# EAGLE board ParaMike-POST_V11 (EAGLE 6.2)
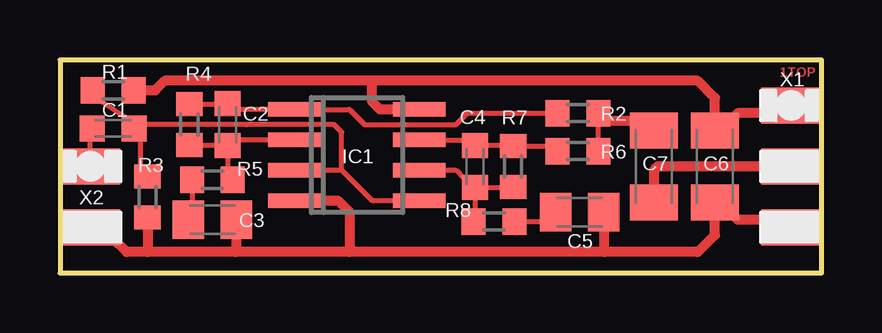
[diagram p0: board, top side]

Size 31.75 x 8.89 mm. Coordinates in mm from the lower left corner, seen from the top.
Outline: 0,8.89 0,0 31.75,0 31.75,8.89 0,8.89
Copper layers (1*16): Top 0.035mm / dielectric 1.5mm / Bottom 0.035mm
Design rules: minimum track width 6mil, minimum drill 12mil, track to track 6mil, track to pad 6mil, pad to pad 6mil, via to via 6mil, smd to smd 6mil, copper to edge 20mil, drill to drill 8mil, minimum pad ring 8mil, minimum via ring 6mil, stop-mask expansion 3mil, vias tented up to drill 0mil, thermal gap 8mil

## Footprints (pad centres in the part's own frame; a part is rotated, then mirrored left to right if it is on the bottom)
C0603K = smd 1.05 x 1.08: 1 -0.875,0; 2 0.875,0
C0805K = smd 1.3 x 1.6: 1 -1,0; 2 1,0
C1206K = smd 1.5 x 2: 1 -1.5,0; 2 1.5,0
SO08 = smd 0.6 x 2.2: 1 -1.905,-2.6; 2 -0.635,-2.6; 3 0.635,-2.6; 4 1.905,-2.6; 5 1.905,2.6; 6 0.635,2.6; 7 -0.635,2.6; 8 -1.905,2.6
R0603 = smd 1 x 1.1: 1 -0.85,0; 2 0.85,0
AKK3PAD-HALF = smd 2.5 x 1.5: 1 0,2.54; 2 0,0; 3 0,-2.54
AKK2PAD-HALF = smd 2.5 x 1.5: 1 0,1.27; 2 0,-1.27

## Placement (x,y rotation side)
C1  22n  [C0603K]  2.22,6.03 0 top
C2  1n  [C0603K]  6.99,6.19 270 top
C3  220n  [C0805K]  6.35,2.22 0 top
C4  1n  [C0603K]  17.3,4.45 270 top
C5  220n  [C0805K]  21.67,2.54 0 top
C6  22u;10V  [C1206K]  27.3,4.45 270 top
C7  22u;10V  [C1206K]  24.77,4.45 270 top
IC1  NJM4556  [SO08]  12.38,4.92 270 top
R1  47k  [R0603]  2.22,7.62 0 top
R2  10E  [R0603]  21.59,6.67 180 top
R3  47k  [R0603]  3.65,3.17 90 top
R4  22k  [R0603]  5.4,6.19 90 top
R5  2k2  [R0603]  6.35,3.89 0 top
R6  10E  [R0603]  21.59,5.08 180 top
R7  22k  [R0603]  18.89,4.45 90 top
R8  2k2  [R0603]  18.1,2.14 180 top
X1  AKK3PAD-HALF  [AKK3PAD-HALF]  30.48,4.45 0 top
X2  AKK2PAD-HALF  [AKK2PAD-HALF]  1.27,3.17 0 top

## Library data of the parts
C1 C2 C4 R1-R8 = rcl
C3 C5 = rcl; SIZE: 0805
C6 C7 = rcl; SIZE: 1206
IC1 = linear
X1 X2 = Akki_V6

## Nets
+BAT: C6.1 IC1.8 R1.2 X1.1
GND: C3.2 C5.2 C6.2 IC1.4 R3.1 X1.3 X2.2
N$1: C3.1 R5.1
N$2: C1.2 IC1.3 IC1.5 R1.1 R3.2
N$3: C2.2 IC1.2 R4.1 R5.2
N$4: C2.1 IC1.1 R2.2 R4.2
N$5: C7.2 X1.2
N$6: C1.1 X2.1
N$7: C7.1 R2.1 R6.1
N$8: C4.2 IC1.6 R7.1 R8.2
N$9: C4.1 IC1.7 R6.2 R7.2
N$10: C5.1 R8.1

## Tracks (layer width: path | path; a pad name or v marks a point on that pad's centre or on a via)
+BAT
  Top 0.406: X1.1 29.84,6.99 29.53,6.67 28.26,6.67 27.94,6.35 27.71,6.35 C6.1 27.3,7.3 26.59,8.02 13.02,8.02 | 13.02,8.02 4.37,8.02 3.97,7.62 R1.2 | IC1.8 13.34,6.83 13.02,7.14 13.02,8.02
GND
  Top 0.406: X1.3 30,1.91 29.53,1.43 29.53,2.22 28.26,2.22 27.94,2.54 27.71,2.54 27.51,2.74 | 22.7,0.87 26.59,0.87 27.3,1.59 27.3,2.54 27.51,2.74 | 22.7,0.87 12.06,0.87 | 12.06,0.87 7.3,0.87 | 7.3,0.87 3.65,0.87 | 3.65,0.87 2.78,0.87 2.22,1.43 1.75,1.43 X2.2 | 27.51,2.74 C6.2 | C3.2 7.35,0.92 7.3,0.87 | R3.1 3.65,0.87 | C5.2 22.67,0.91 22.7,0.87 | IC1.4 11.59,3.02 12.06,2.54 12.06,0.87
N$1
  Top 0.203: R5.1 5.5,2.37 C3.1
N$2
  Top 0.203: C1.2 3.1,6.11 2.7,6.51 1.75,7.14 1.37,7.52 R1.1 | C1.2 3.1,5.95 3.33,5.71 3.33,4.34 R3.2 | IC1.3 11.75,4.29 | 11.75,4.29 13.02,3.02 IC1.5 | 11.75,4.29 11.75,5.87 11.43,6.19 7.78,6.19 3.26,6.19 C1.2
N$3
  Top 0.203: 7.22,5.08 C2.2 | R4.1 6.96,5.34 C2.2 | C2.2 6.99,4.1 R5.2 | IC1.2 7.22,5.56 C2.2
N$4
  Top 0.203: R4.2 6.96,7.04 C2.1 7.18,6.87 | 7.38,6.67 7.18,6.87 | 7.18,6.87 7.34,6.83 IC1.1 12.06,6.83 12.7,6.19 16.51,6.19 16.99,6.67 R2.2 20.42,6.35
N$5
  Top 0.406: X1.2 24.92,4.45 24.77,4.29 C7.2
N$6
  Top 0.203: X2.1 1.27,5.96 C1.1
N$7
  Top 0.203: R6.1 R2.1
  Top 0.406: C7.1 24.36,6.35 22.7,6.35 22.44,6.61 R2.1
N$8
  Top 0.203: C4.2 17.3,2.04 R8.2 | 18.87,3.73 R7.1 18.87,3.57 C4.2 | IC1.6 16.51,4.29 16.83,3.97 16.91,3.97 C4.2
N$9
  Top 0.203: 17.06,5.08 C4.1 | R7.2 18.87,5.32 C4.1 | 18.87,5.48 R7.2 | C4.1 17.23,5.56 IC1.7 | R7.2 20.52,5.29 R6.2
N$10
  Top 0.203: 20.27,1.98 20.35,2.09 | 20.35,2.09 C5.1 | R8.1 20.29,2.14 20.35,2.09

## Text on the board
Top: 1TOP
tDocu: (c) ASkr | ParaMike V1.1 | POST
